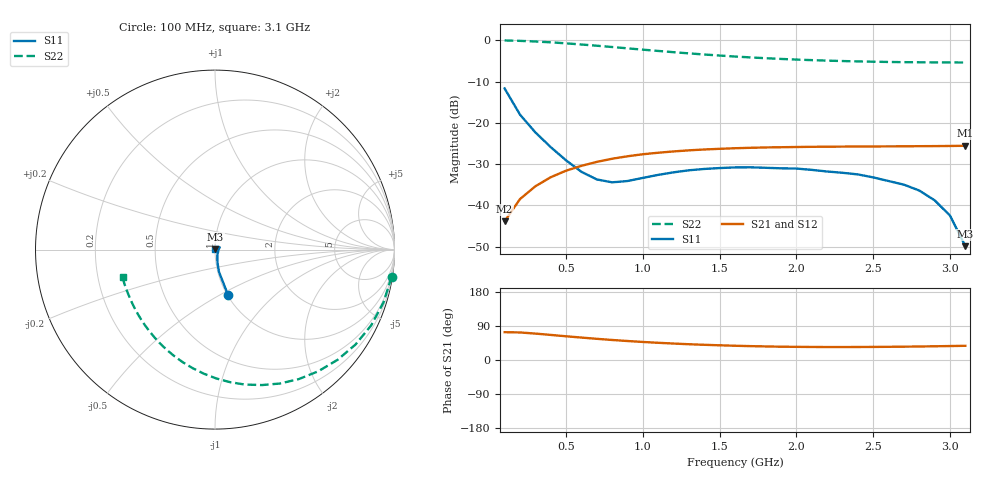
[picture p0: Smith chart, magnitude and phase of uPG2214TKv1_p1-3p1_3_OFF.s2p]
! NEC Compound Semiconductor Devices Ltd.
! 4.February 2005
! uPG2214TK
! Vcont1=3.0v Vcont2=0v / IN-OUT1 ( OFF )
! OUT2:50ohm termination
#  GHz  S  MA  R  50
!  f  S11  S21  S12  S22
!  GHz  MAG  ANG  MAG  ANG  MAG  ANG  MAG  ANG
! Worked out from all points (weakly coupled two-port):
!   31 points, 100 MHz to 3.1 GHz, reference 50 ohm
!   highest |S21| = -25.56 dB at 3.1 GHz (marker M1); lowest = -43.9 dB at 100 MHz (marker M2)
!   lowest |S11| = -49.9 dB at 3.1 GHz (marker M3), VSWR 1.01, Z = 50.3 + j0.192 ohm
!   |S11| at or under -10 dB: start of sweep to end of sweep
!   |S22| runs from -5.4 to 0.0 dB; largest |S21 - S12| = 0.00029
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0.1  0.2607 -74.0  0.0064 73.4  0.0064 73.2  0.9953 -8.8
0.2  0.1258 -79.9  0.0119 72.7  0.0118 72.9  0.984 -17.4
0.3  0.0766 -79.4  0.017 69.7  0.017 69.8  0.9671 -25.9
0.4  0.0508 -75.3  0.0219 66.2  0.0218 66.4  0.9446 -34.1
0.5  0.0351 -67.5  0.0263 62.6  0.0263 62.6  0.9182 -42.0
0.6  0.0255 -54.4  0.0301 59.2  0.0302 59.0  0.8891 -49.7
0.7  0.0206 -36.7  0.0336 55.9  0.0336 55.7  0.8593 -57.1
0.8  0.019 -18.3  0.0367 52.8  0.0366 52.7  0.8289 -64.2
0.9  0.0197 -2.9  0.0393 50.1  0.0392 50.0  0.7987 -70.9
1.1  0.0234 13.6  0.0434 45.4  0.0434 45.3  0.743 -83.6
1.3  0.0266 20.5  0.0464 41.6  0.0463 41.6  0.694 -95.2
1.6  0.0288 25.5  0.0492 37.6  0.0492 37.5  0.6357 -110.8
1.8  0.0285 28.1  0.0503 35.8  0.0501 35.8  0.6065 -120.1
2  0.0279 32.2  0.0509 34.7  0.0508 34.7  0.5837 -128.6
2.1  0.0269 33.4  0.0512 34.4  0.051 34.4  0.5749 -132.6
2.4  0.0237 40.6  0.0516 34.3  0.0517 34.0  0.5548 -143.5
2.6  0.0197 45.1  0.0518 34.8  0.0516 34.8  0.5462 -149.9
2.7  0.0178 47.2  0.0519 35.2  0.0517 35.3  0.5433 -152.9
2.8  0.0151 47.2  0.0521 35.6  0.0519 35.8  0.5413 -155.7
2.9  0.0115 47.0  0.0522 36.2  0.0521 36.4  0.5399 -158.4
3  0.0075 46.9  0.0524 36.8  0.0524 37.0  0.5388 -161.0
3.1  0.0032 36.7  0.0527 37.5  0.0527 37.6  0.5377 -163.4
